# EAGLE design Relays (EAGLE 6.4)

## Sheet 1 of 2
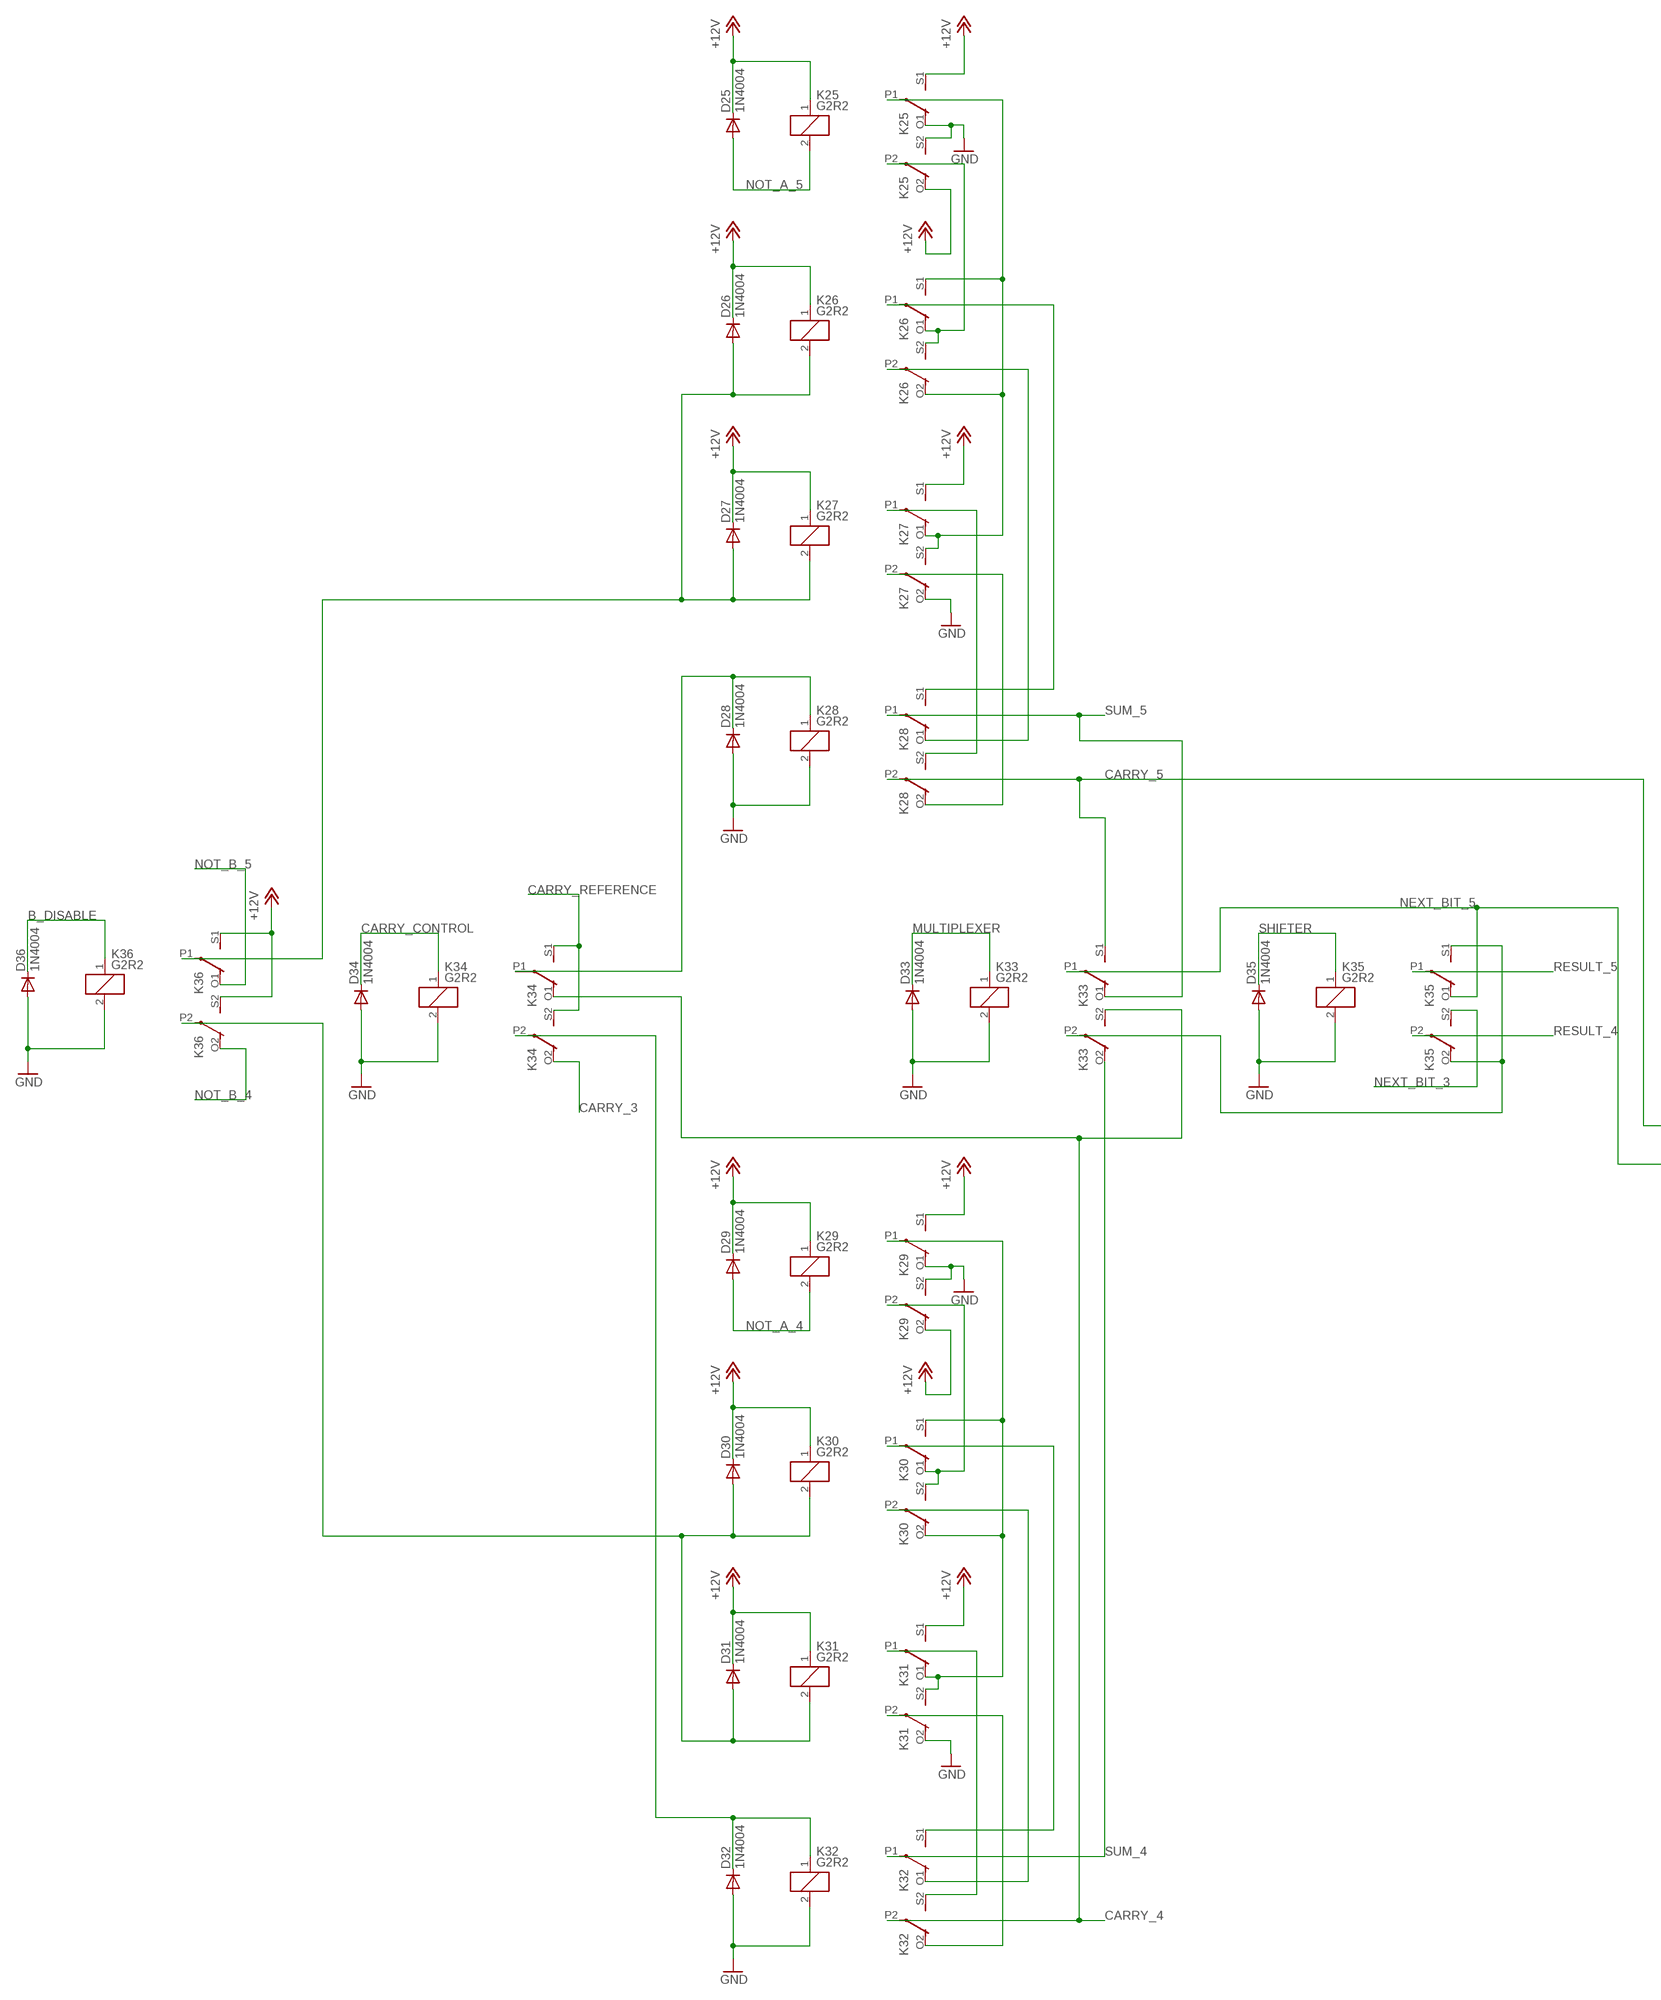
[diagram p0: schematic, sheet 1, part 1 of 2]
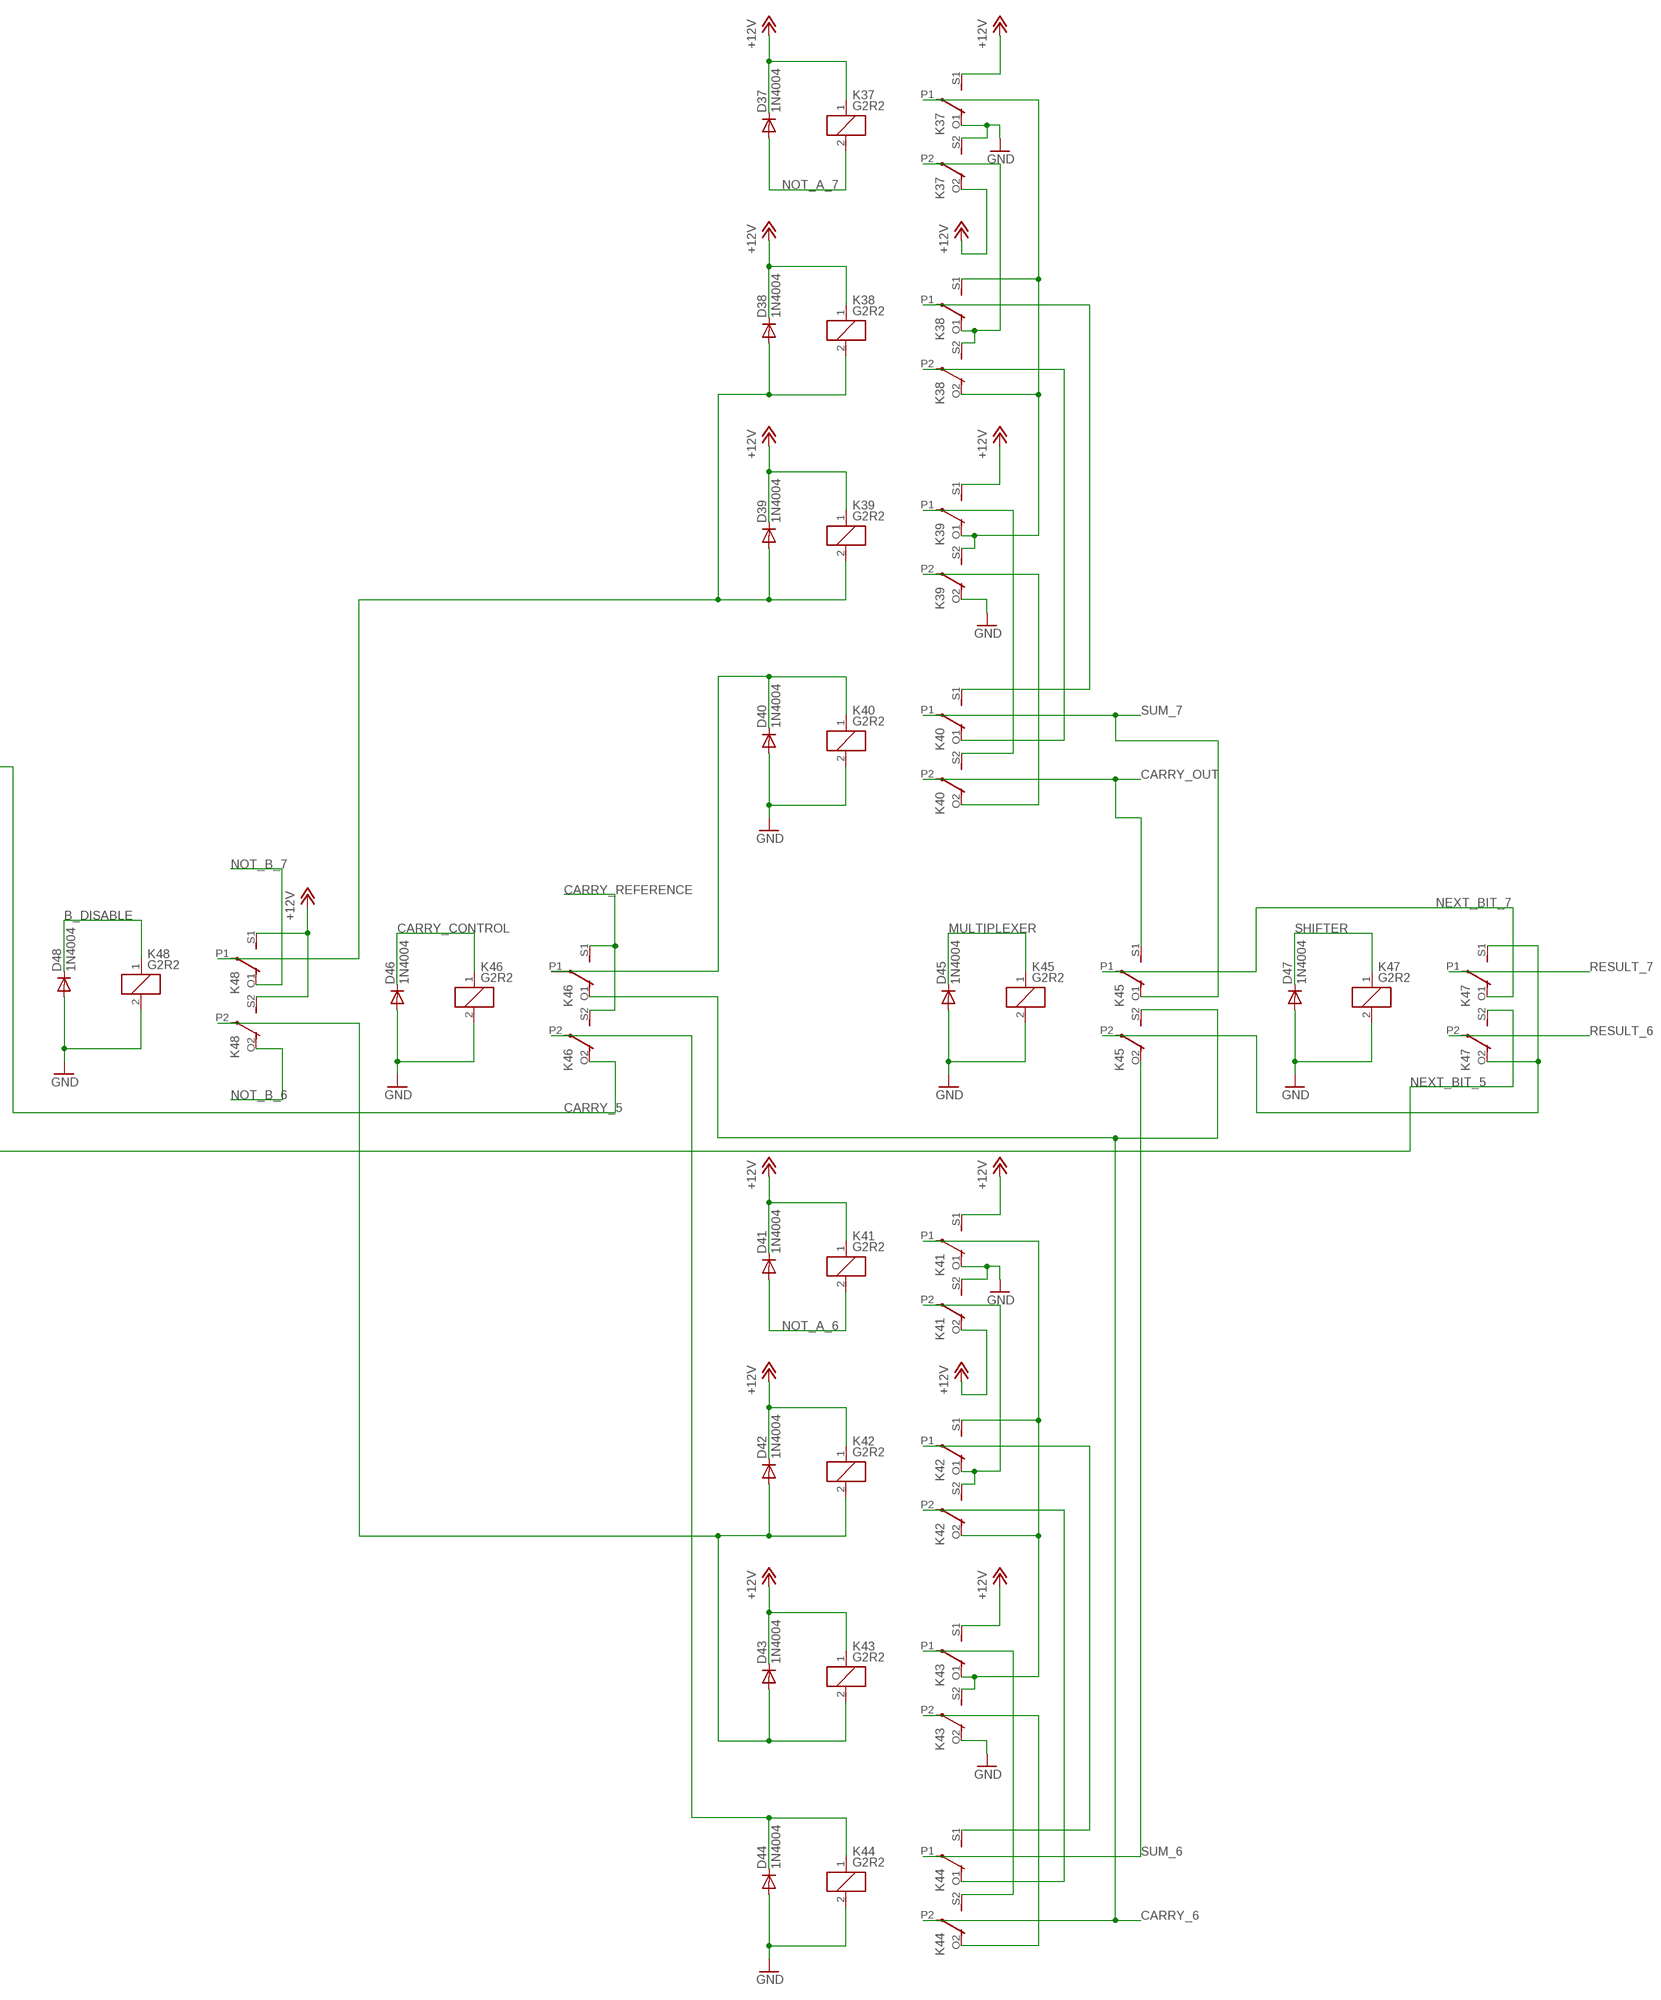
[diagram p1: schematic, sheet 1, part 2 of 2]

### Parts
D25  1N4004  [DO41-10]
D26  1N4004  [DO41-10]
D27  1N4004  [DO41-10]
D28  1N4004  [DO41-10]
D29  1N4004  [DO41-10]
D30  1N4004  [DO41-10]
D31  1N4004  [DO41-10]
D32  1N4004  [DO41-10]
D33  1N4004  [DO41-10]
D34  1N4004  [DO41-10]
D35  1N4004  [DO41-10]
D36  1N4004  [DO41-10]
D37  1N4004  [DO41-10]
D38  1N4004  [DO41-10]
D39  1N4004  [DO41-10]
D40  1N4004  [DO41-10]
D41  1N4004  [DO41-10]
D42  1N4004  [DO41-10]
D43  1N4004  [DO41-10]
D44  1N4004  [DO41-10]
D45  1N4004  [DO41-10]
D46  1N4004  [DO41-10]
D47  1N4004  [DO41-10]
D48  1N4004  [DO41-10]
K25  G2R2  [G2R2]
K26  G2R2  [G2R2]
K27  G2R2  [G2R2]
K28  G2R2  [G2R2]
K29  G2R2  [G2R2]
K30  G2R2  [G2R2]
K31  G2R2  [G2R2]
K32  G2R2  [G2R2]
K33  G2R2  [G2R2]
K34  G2R2  [G2R2]
K35  G2R2  [G2R2]
K36  G2R2  [G2R2]
K37  G2R2  [G2R2]
K38  G2R2  [G2R2]
K39  G2R2  [G2R2]
K40  G2R2  [G2R2]
K41  G2R2  [G2R2]
K42  G2R2  [G2R2]
K43  G2R2  [G2R2]
K44  G2R2  [G2R2]
K45  G2R2  [G2R2]
K46  G2R2  [G2R2]
K47  G2R2  [G2R2]
K48  G2R2  [G2R2]

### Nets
+12V [12V_Power]: D25.C D26.C D27.C D29.C D30.C D31.C D37.C D38.C D39.C D41.C D42.C D43.C K25.1 K25.O2(3:O) K25.S1(2:S) K26.1 K27.1 K27.S1(2:S) K29.1 K29.O2(3:O) K29.S1(2:S) K30.1 K31.1 K31.S1(2:S) K36.S1(2:S) K36.S2(3:S) K37.1 K37.O2(3:O) K37.S1(2:S) K38.1 K39.1 K39.S1(2:S) K41.1 K41.O2(3:O) K41.S1(2:S) K42.1 K43.1 K43.S1(2:S) K48.S1(2:S) K48.S2(3:S) ; also sheet 2
B_DISABLE [Relay_Interconnects]: D36.C D48.C K36.1 K48.1 ; also sheet 2
CARRY_3: K34.O2(3:O) ; also sheet 2
CARRY_4: K32.P2(3:P) K33.S2(3:S) K34.O1(2:O)
CARRY_5: K28.P2(3:P) K33.S1(2:S) K46.O2(3:O)
CARRY_6: K44.P2(3:P) K45.S2(3:S) K46.O1(2:O)
CARRY_CONTROL [Relay_Interconnects]: D34.C D46.C K34.1 K46.1 ; also sheet 2
CARRY_OUT [Relay_Interconnects]: K40.P2(3:P) K45.S1(2:S) ; also sheet 2
CARRY_REFERENCE [Relay_Interconnects]: K34.S1(2:S) K34.S2(3:S) K46.S1(2:S) K46.S2(3:S) ; also sheet 2
GND [Ground]: D28.A D32.A D33.A D34.A D35.A D36.A D40.A D44.A D45.A D46.A D47.A D48.A K25.O1(2:O) K25.S2(3:S) K27.O2(3:O) K28.2 K29.O1(2:O) K29.S2(3:S) K31.O2(3:O) K32.2 K33.2 K34.2 K35.2 K36.2 K37.O1(2:O) K37.S2(3:S) K39.O2(3:O) K40.2 K41.O1(2:O) K41.S2(3:S) K43.O2(3:O) K44.2 K45.2 K46.2 K47.2 K48.2 ; also sheet 2
MULTIPLEXER [Relay_Interconnects]: D33.C D45.C K33.1 K45.1 ; also sheet 2
N$37: D28.C K28.1 K34.P1(2:P)
N$38: K25.P2(3:P) K26.O1(2:O) K26.S2(3:S)
N$39: K25.P1(2:P) K26.O2(3:O) K26.S1(2:S) K27.O1(2:O) K27.S2(3:S)
N$40: K27.P2(3:P) K28.O2(3:O)
N$41: K27.P1(2:P) K28.S2(3:S)
N$42: K26.P2(3:P) K28.O1(2:O)
N$43: K26.P1(2:P) K28.S1(2:S)
N$44: D32.C K32.1 K34.P2(3:P)
N$45: K29.P2(3:P) K30.O1(2:O) K30.S2(3:S)
N$46: K29.P1(2:P) K30.O2(3:O) K30.S1(2:S) K31.O1(2:O) K31.S2(3:S)
N$47: K31.P2(3:P) K32.O2(3:O)
N$48: K31.P1(2:P) K32.S2(3:S)
N$49: K30.P2(3:P) K32.O1(2:O)
N$50: K30.P1(2:P) K32.S1(2:S)
N$51: D26.A D27.A K26.2 K27.2 K36.P1(2:P)
N$52: D30.A D31.A K30.2 K31.2 K36.P2(3:P)
N$53: K33.P2(3:P) K35.O2(3:O) K35.S1(2:S)
N$54: D40.C K40.1 K46.P1(2:P)
N$55: K37.P2(3:P) K38.O1(2:O) K38.S2(3:S)
N$56: K37.P1(2:P) K38.O2(3:O) K38.S1(2:S) K39.O1(2:O) K39.S2(3:S)
N$57: K39.P2(3:P) K40.O2(3:O)
N$58: K39.P1(2:P) K40.S2(3:S)
N$59: K38.P2(3:P) K40.O1(2:O)
N$60: K38.P1(2:P) K40.S1(2:S)
N$61: D44.C K44.1 K46.P2(3:P)
N$62: K41.P2(3:P) K42.O1(2:O) K42.S2(3:S)
N$63: K41.P1(2:P) K42.O2(3:O) K42.S1(2:S) K43.O1(2:O) K43.S2(3:S)
N$64: K43.P2(3:P) K44.O2(3:O)
N$65: K43.P1(2:P) K44.S2(3:S)
N$66: K42.P2(3:P) K44.O1(2:O)
N$67: K42.P1(2:P) K44.S1(2:S)
N$68: D38.A D39.A K38.2 K39.2 K48.P1(2:P)
N$69: D42.A D43.A K42.2 K43.2 K48.P2(3:P)
N$70: K45.P2(3:P) K47.O2(3:O) K47.S1(2:S)
NEXT_BIT_3 [Relay_Interconnects]: K35.S2(3:S) ; also sheet 2
NEXT_BIT_5: K33.P1(2:P) K35.O1(2:O) K47.S2(3:S)
NEXT_BIT_7 [Relay_Interconnects]: K45.P1(2:P) K47.O1(2:O) ; also sheet 2
NOT_A_4 [Relay_Interconnects]: D29.A K29.2 ; also sheet 2
NOT_A_5 [Relay_Interconnects]: D25.A K25.2 ; also sheet 2
NOT_A_6 [Relay_Interconnects]: D41.A K41.2 ; also sheet 2
NOT_A_7 [Relay_Interconnects]: D37.A K37.2 ; also sheet 2
NOT_B_4 [Relay_Interconnects]: K36.O2(3:O) ; also sheet 2
NOT_B_5 [Relay_Interconnects]: K36.O1(2:O) ; also sheet 2
NOT_B_6 [Relay_Interconnects]: K48.O2(3:O) ; also sheet 2
NOT_B_7 [Relay_Interconnects]: K48.O1(2:O) ; also sheet 2
RESULT_4 [Relay_Interconnects]: K35.P2(3:P) ; also sheet 2
RESULT_5 [Relay_Interconnects]: K35.P1(2:P) ; also sheet 2
RESULT_6 [Relay_Interconnects]: K47.P2(3:P) ; also sheet 2
RESULT_7 [Relay_Interconnects]: K47.P1(2:P) ; also sheet 2
SHIFTER [Relay_Interconnects]: D35.C D47.C K35.1 K47.1 ; also sheet 2
SUM_4: K32.P1(2:P) K33.O2(3:O)
SUM_5: K28.P1(2:P) K33.O1(2:O)
SUM_6: K44.P1(2:P) K45.O2(3:O)
SUM_7: K40.P1(2:P) K45.O1(2:O)

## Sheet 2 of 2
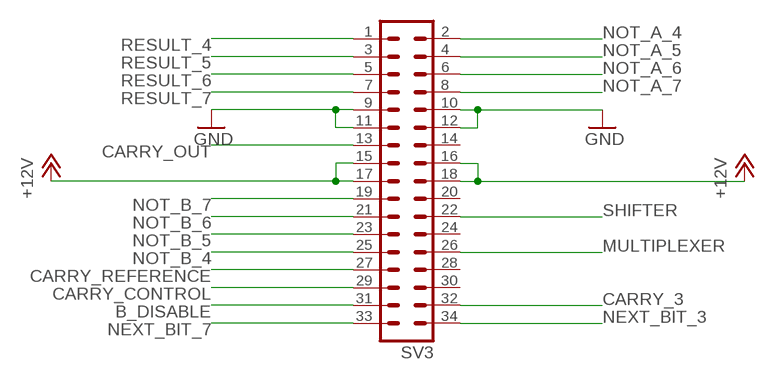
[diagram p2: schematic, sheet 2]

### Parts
SV3  ML34  [ML34]

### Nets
+12V [12V_Power]: SV3.15 SV3.16 SV3.17 SV3.18 ; also sheet 1
B_DISABLE [Relay_Interconnects]: SV3.31 ; also sheet 1
CARRY_3: SV3.32 ; also sheet 1
CARRY_CONTROL [Relay_Interconnects]: SV3.29 ; also sheet 1
CARRY_OUT [Relay_Interconnects]: SV3.13 ; also sheet 1
CARRY_REFERENCE [Relay_Interconnects]: SV3.27 ; also sheet 1
GND [Ground]: SV3.9 SV3.10 SV3.11 SV3.12 ; also sheet 1
MULTIPLEXER [Relay_Interconnects]: SV3.26 ; also sheet 1
NEXT_BIT_3 [Relay_Interconnects]: SV3.34 ; also sheet 1
NEXT_BIT_7 [Relay_Interconnects]: SV3.33 ; also sheet 1
NOT_A_4 [Relay_Interconnects]: SV3.2 ; also sheet 1
NOT_A_5 [Relay_Interconnects]: SV3.4 ; also sheet 1
NOT_A_6 [Relay_Interconnects]: SV3.6 ; also sheet 1
NOT_A_7 [Relay_Interconnects]: SV3.8 ; also sheet 1
NOT_B_4 [Relay_Interconnects]: SV3.25 ; also sheet 1
NOT_B_5 [Relay_Interconnects]: SV3.23 ; also sheet 1
NOT_B_6 [Relay_Interconnects]: SV3.21 ; also sheet 1
NOT_B_7 [Relay_Interconnects]: SV3.19 ; also sheet 1
RESULT_4 [Relay_Interconnects]: SV3.1 ; also sheet 1
RESULT_5 [Relay_Interconnects]: SV3.3 ; also sheet 1
RESULT_6 [Relay_Interconnects]: SV3.5 ; also sheet 1
RESULT_7 [Relay_Interconnects]: SV3.7 ; also sheet 1
SHIFTER [Relay_Interconnects]: SV3.22 ; also sheet 1
Unconnected: SV3.14 SV3.20 SV3.24 SV3.28 SV3.30

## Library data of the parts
D25-D48 = diode:1N4004: DIODE
K25-K48 = relay:G2R2: RELAY 2 x switch, Omron; MF: OMRON COMPONENTS USA; MPN: G2R-2-DC6; OC_FARNELL: unknown; OC_NEWARK: 89C5317
SV3 = con-harting-ml:ML34: HARTING; OC_FARNELL: unknown; OC_NEWARK: unknown

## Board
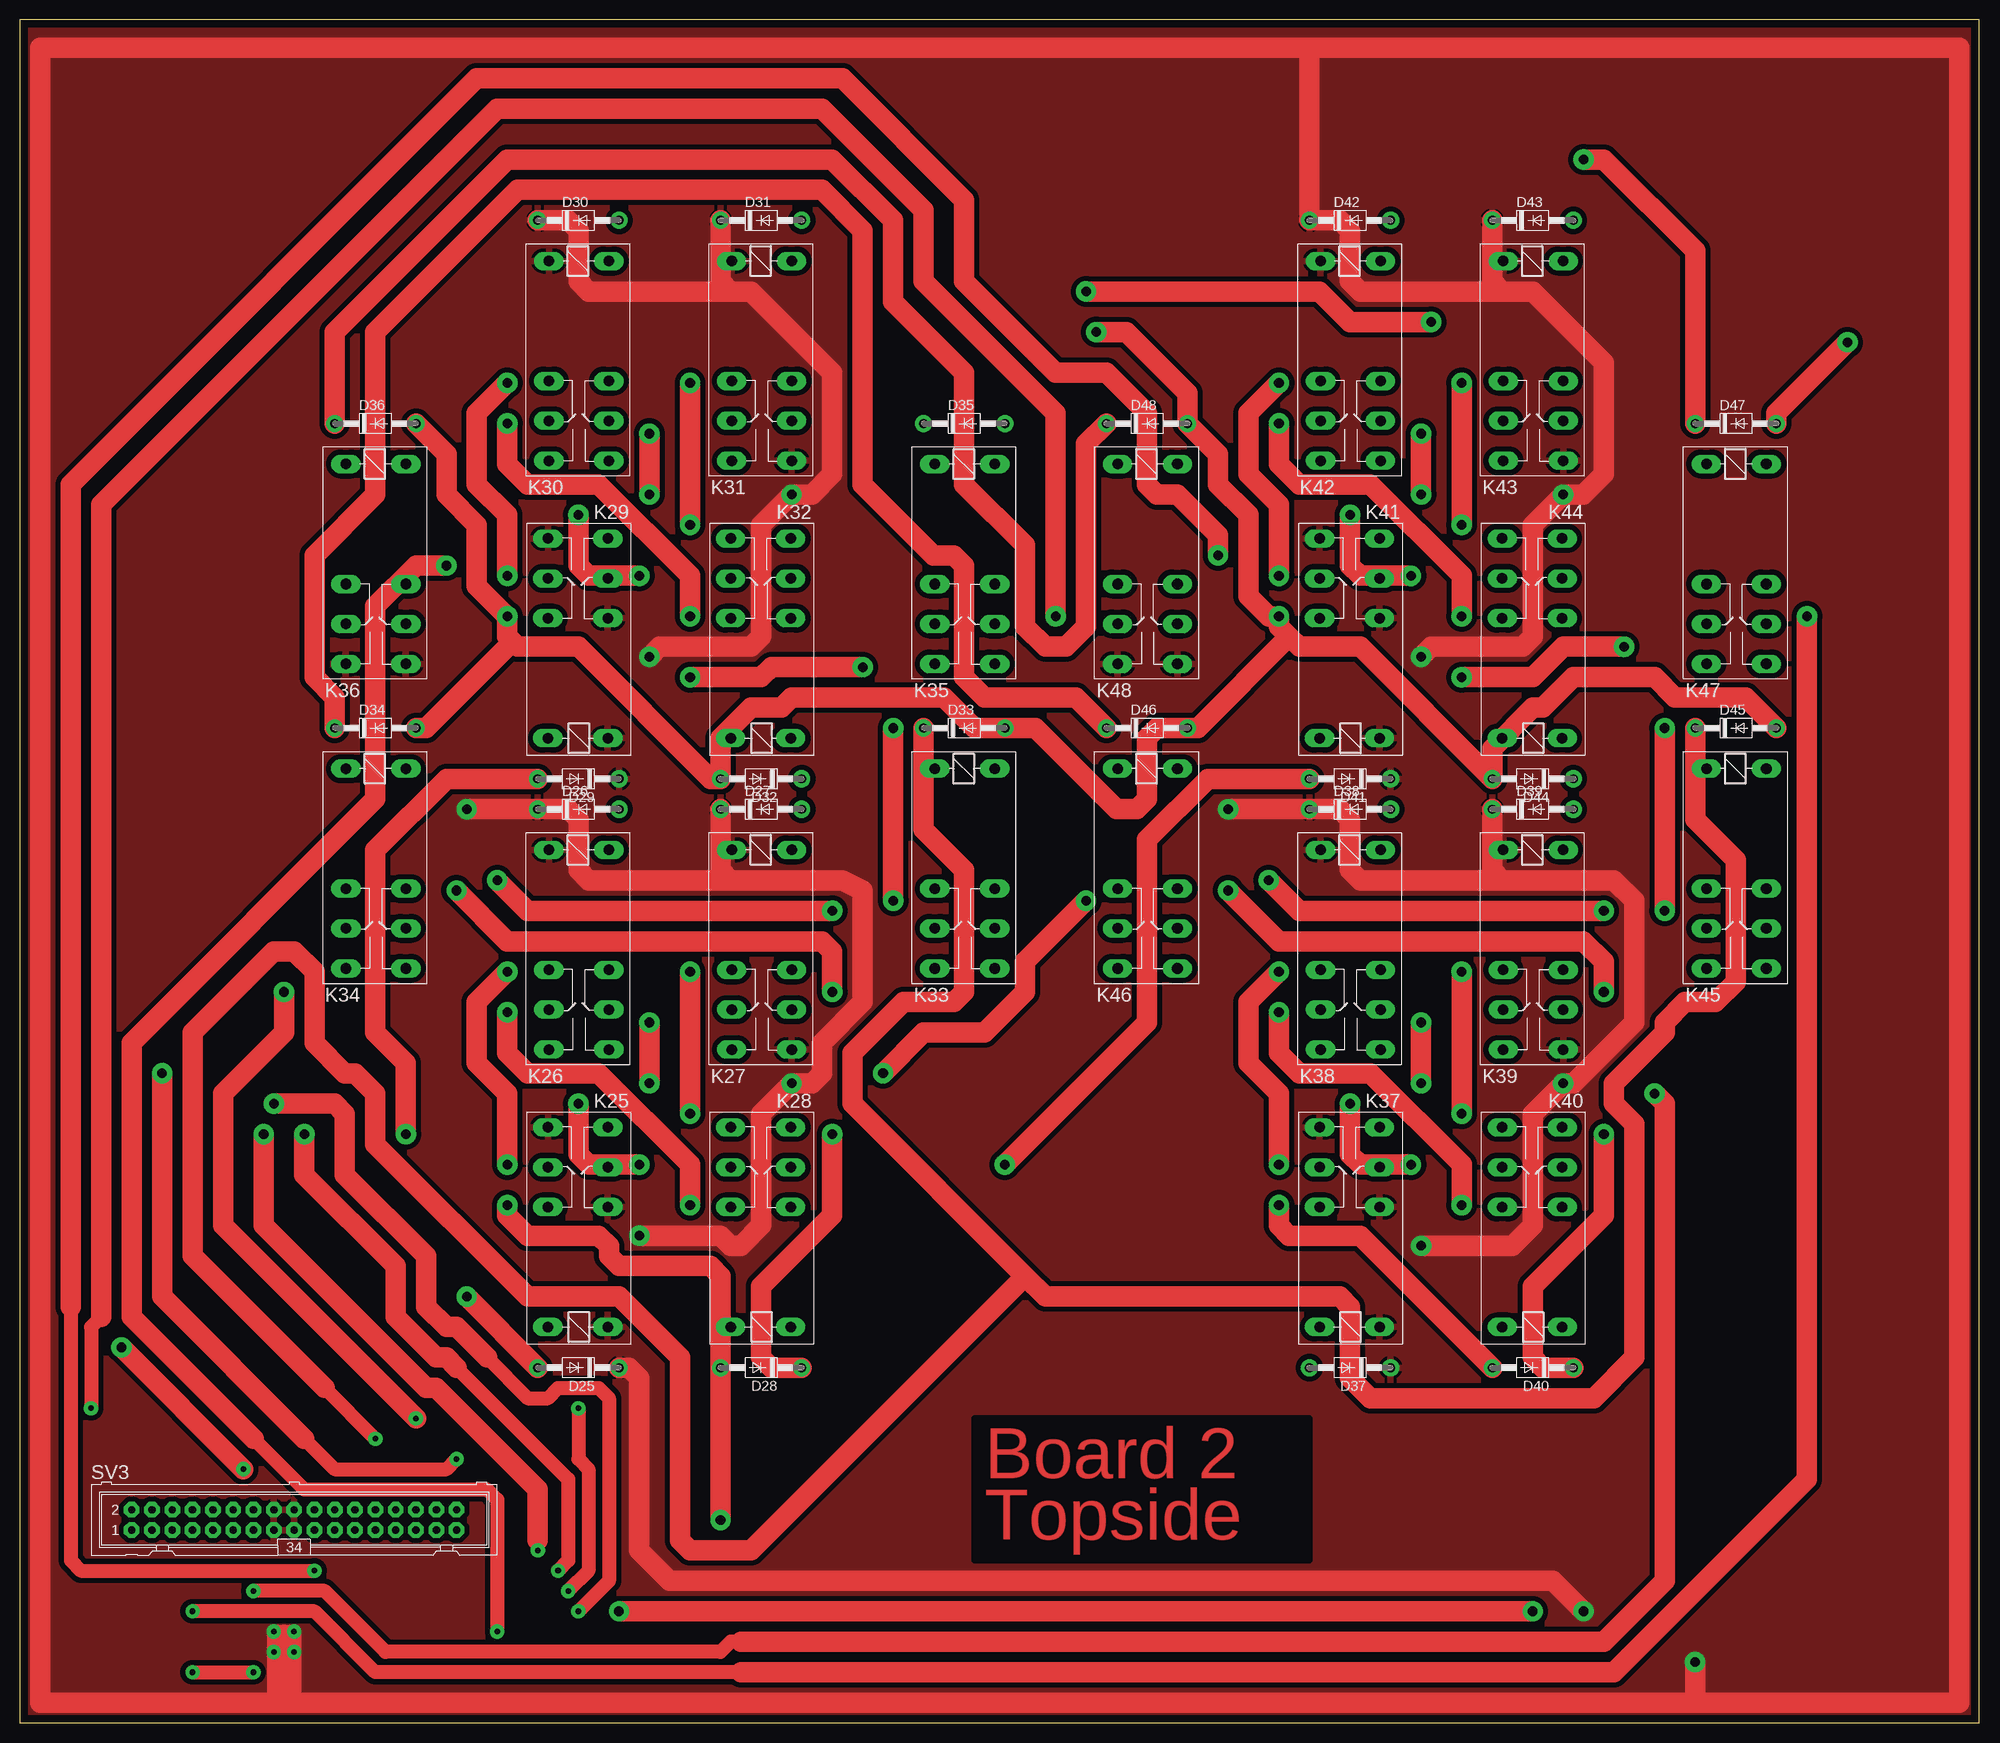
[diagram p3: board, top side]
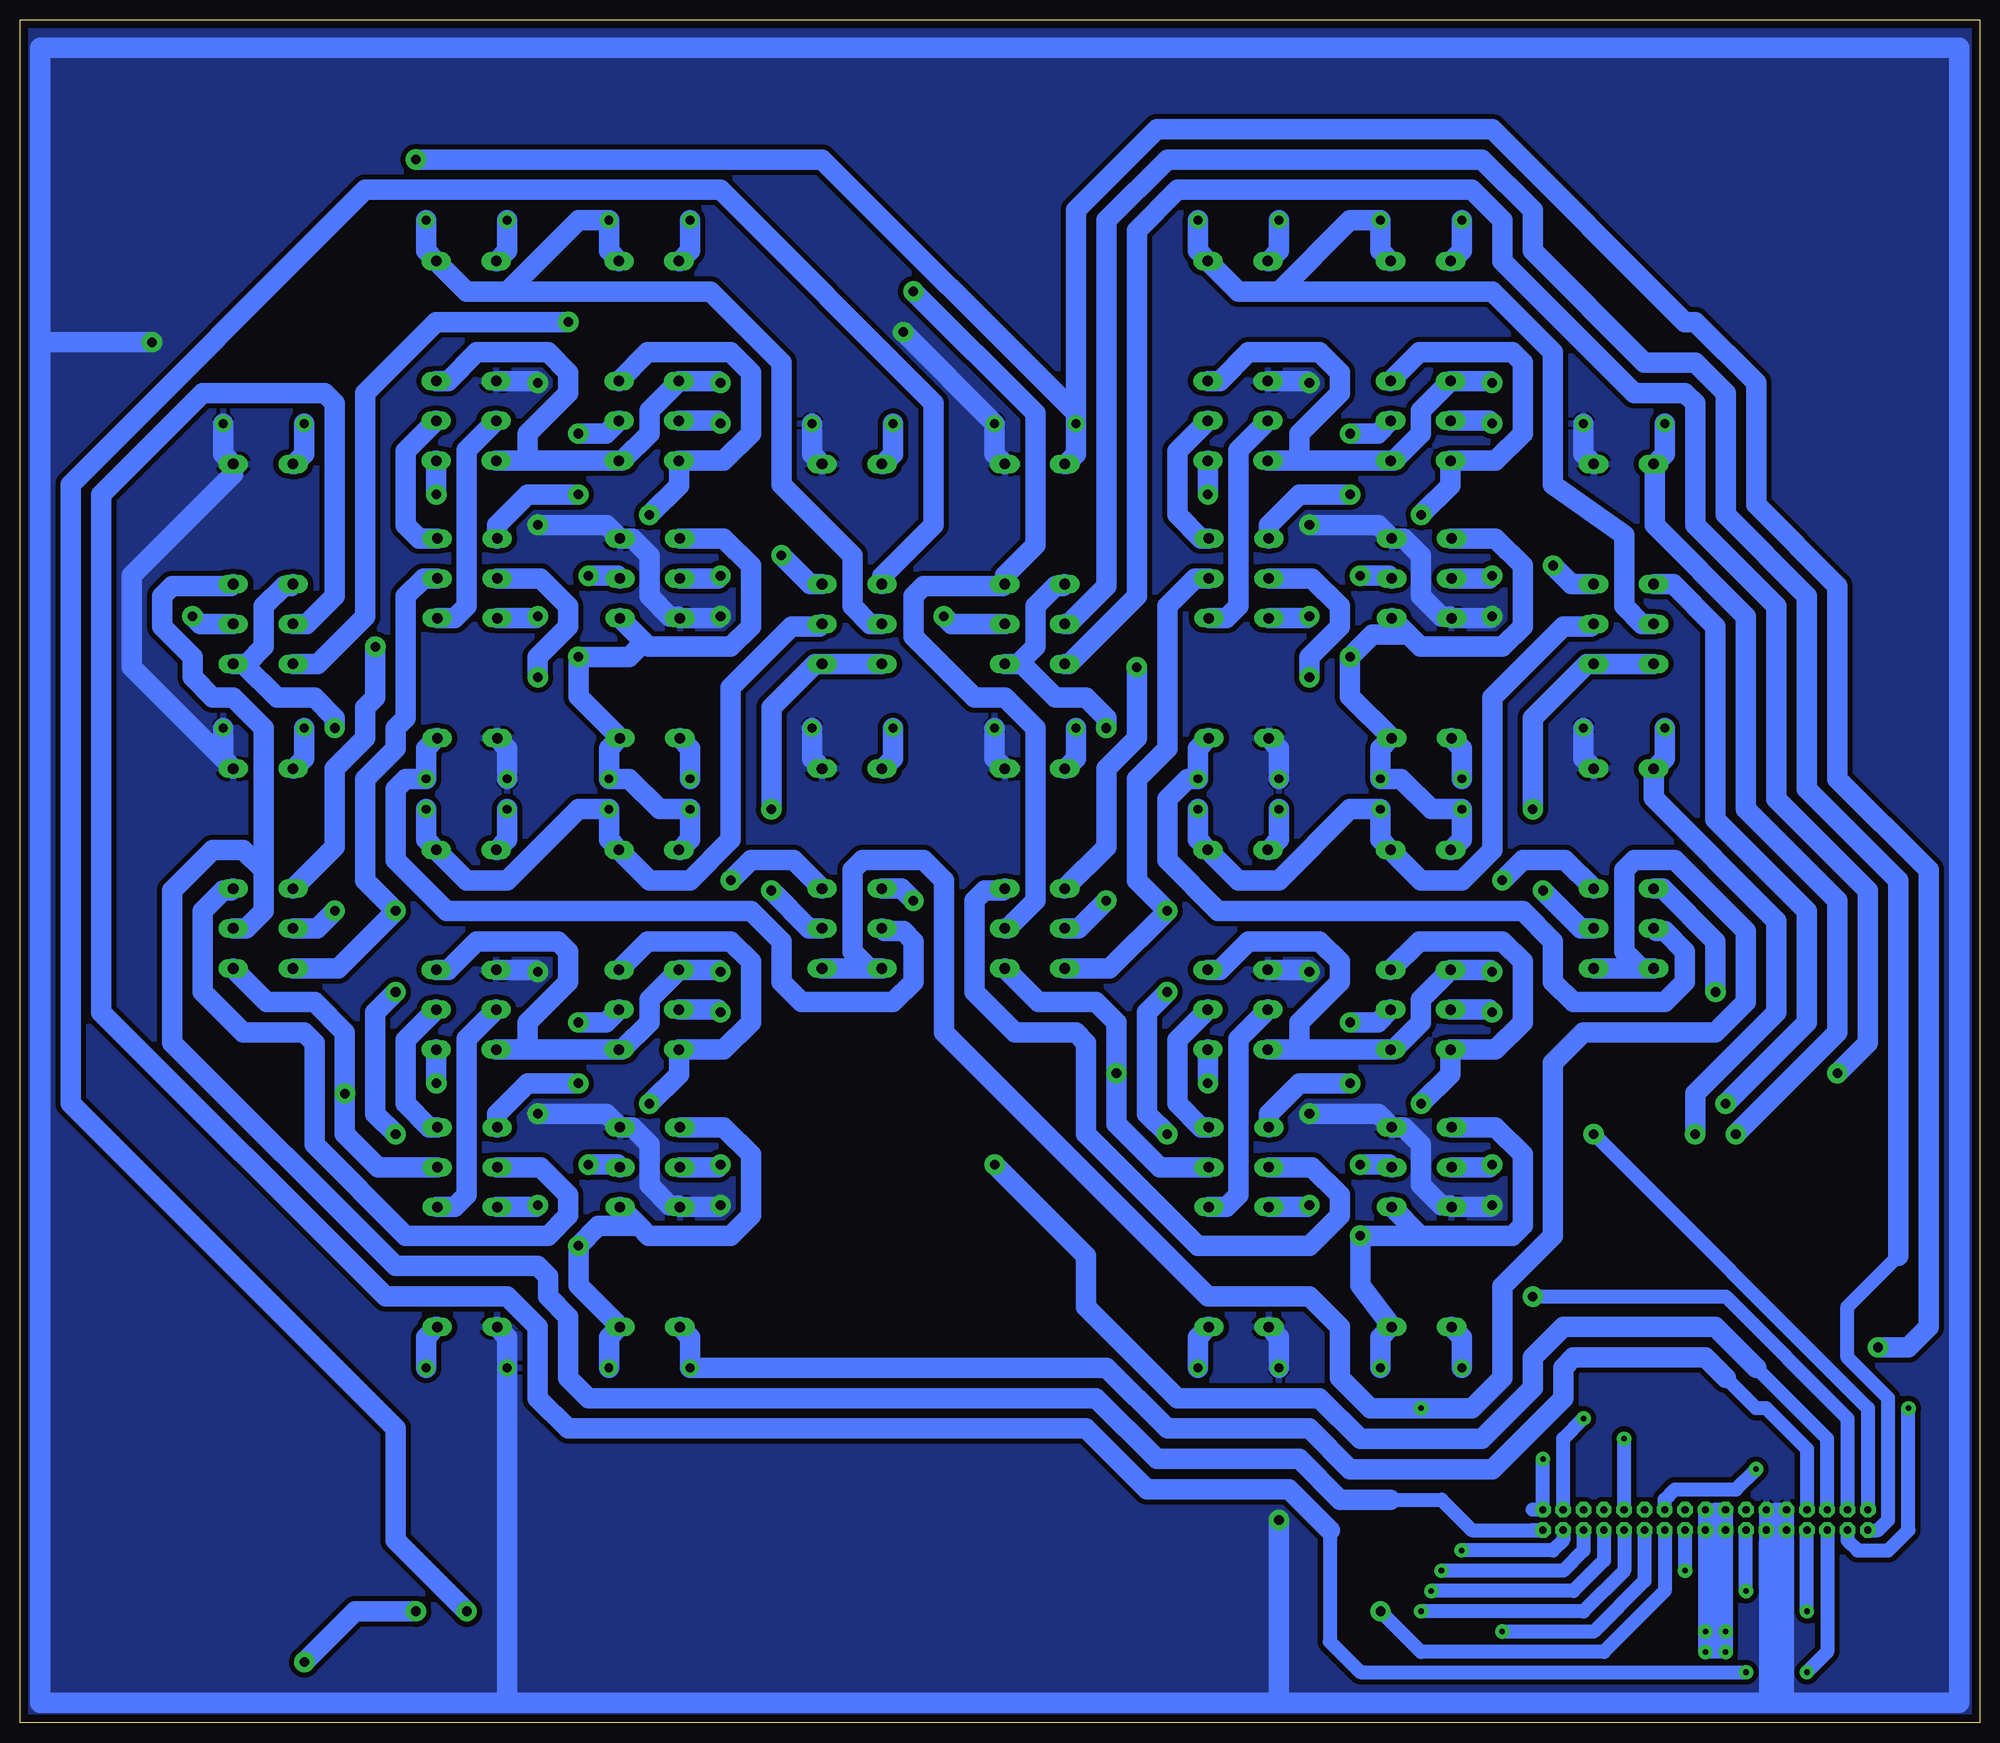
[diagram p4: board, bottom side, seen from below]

Size 245.09 x 213.03 mm. Coordinates in mm from the lower left corner, seen from the top.
Outline: 0,0 245.09,0 245.09,213.03 0,213.03 0,0
Copper layers (1*16): Top 0.035mm / dielectric 1.5mm / Bottom 0.035mm
Design rules "arm-rules-modified": minimum track width 20mil, minimum drill 24mil, track to track 25mil, track to pad 20mil, pad to pad 15mil, via to via 20mil, smd to smd 8mil, copper to edge 40mil, drill to drill 12mil, minimum pad ring 20mil, minimum via ring 20mil, stop-mask expansion 0mil, vias tented up to drill 0mil, thermal gap 15mil

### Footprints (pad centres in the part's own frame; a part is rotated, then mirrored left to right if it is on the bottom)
DO41-10 = drill 1.118: A 5.08,0; C -5.08,0
G2R2 = drill 1.321 long: 1 -2.54,-3.683; 2 -2.54,3.81; O1 12.471,3.81; O2 12.471,-3.683; P1 17.45,3.81; P2 17.45,-3.683; S1 22.454,3.81; S2 22.454,-3.683
ML34 = drill 0.914 octagon: 1 -20.32,-1.27; 2 -20.32,1.27; 3 -17.78,-1.27; 4 -17.78,1.27; 5 -15.24,-1.27; 6 -15.24,1.27; 7 -12.7,-1.27; 8 -12.7,1.27; 9 -10.16,-1.27; 10 -10.16,1.27; 11 -7.62,-1.27; 12 -7.62,1.27; 13 -5.08,-1.27; 14 -5.08,1.27; 15 -2.54,-1.27; 16 -2.54,1.27; 17 0,-1.27; 18 0,1.27; 19 2.54,-1.27; 20 2.54,1.27; 21 5.08,-1.27; 22 5.08,1.27; 23 7.62,-1.27; 24 7.62,1.27; 25 10.16,-1.27; 26 10.16,1.27; 27 12.7,-1.27; 28 12.7,1.27; 29 15.24,-1.27; 30 15.24,1.27; 31 17.78,-1.27; 32 17.78,1.27; 33 20.32,-1.27; 34 20.32,1.27

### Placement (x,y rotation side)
D25  69.85,44.45 180 top
D26  69.85,114.3 0 top
D27  92.71,114.3 0 top
D28  92.71,44.45 180 top
D29  69.85,118.11 180 top
D30  69.85,187.96 0 top
D31  92.71,187.96 0 top
D32  92.71,118.11 180 top
D33  118.11,124.46 0 top
D34  44.45,124.46 0 top
D35  118.11,162.56 0 top
D36  44.45,162.56 0 top
D37  166.37,44.45 180 top
D38  166.37,114.3 0 top
D39  189.23,114.3 0 top
D40  189.23,44.45 180 top
D41  166.37,118.11 180 top
D42  166.37,187.96 0 top
D43  189.23,187.96 0 top
D44  189.23,118.11 180 top
D45  214.63,124.46 0 top
D46  140.97,124.46 0 top
D47  214.63,162.56 0 top
D48  140.97,162.56 0 top
K25  69.85,52.07 90 top
K26  69.85,106.68 270 top
K27  92.71,106.68 270 top
K28  92.71,52.07 90 top
K29  69.85,125.73 90 top
K30  69.85,180.34 270 top
K31  92.71,180.34 270 top
K32  92.71,125.73 90 top
K33  118.11,116.84 270 top
K34  44.45,116.84 270 top
K35  118.11,154.94 270 top
K36  44.45,154.94 270 top
K37  166.37,52.07 90 top
K38  166.37,106.68 270 top
K39  189.23,106.68 270 top
K40  189.23,52.07 90 top
K41  166.37,125.73 90 top
K42  166.37,180.34 270 top
K43  189.23,180.34 270 top
K44  189.23,125.73 90 top
K45  214.63,116.84 270 top
K46  140.97,116.84 270 top
K47  214.63,154.94 270 top
K48  140.97,154.94 270 top
SV3  34.29,25.4 0 top

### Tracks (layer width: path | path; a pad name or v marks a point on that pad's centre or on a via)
+12V  (via drill 0.7 pad 1.78, 1.2 pad 2.54)
  Top 1.778: 31.75,2.54 v31.75,11.43 33.02,11.43 | 33.02,11.43 v34.29,11.43 v34.29,8.89 34.29,2.54 | 33.02,11.43 33.02,2.54
  Top 2.54: v175.26,59.69 186.69,59.69 189.23,62.23 189.23,76.2 v193.04,80.01 194.31,80.01 201.93,87.63 201.93,102.87 199.39,105.41 185.42,105.41 | 185.42,179.07 189.23,179.07 198.12,170.18 198.12,156.21 195.58,153.67 v193.04,153.67 189.23,149.86 189.23,135.89 187.96,134.62 176.53,134.62 v175.26,133.35 | 185.42,179.07 184.15,180.34 D43.C | 88.9,105.41 102.87,105.41 105.41,104.14 105.41,90.17 100.33,85.09 100.33,81.28 99.06,80.01 v96.52,80.01 92.71,76.2 92.71,62.23 90.17,59.69 88.9,59.69 87.63,60.96 v77.47,60.96 | 88.9,105.41 87.63,106.68 D27.C | 88.9,179.07 91.44,179.07 101.6,168.91 101.6,156.21 99.06,153.67 v96.52,153.67 92.71,149.86 92.71,135.89 91.44,134.62 80.01,134.62 v78.74,133.35 | 88.9,179.07 87.63,180.34 D31.C | 185.42,105.41 184.15,106.68 D39.C | 88.9,105.41 71.12,105.41 69.85,106.68 69.85,113.03 68.58,114.3 D26.C v55.88,114.3 | 88.9,179.07 71.12,179.07 69.85,180.34 69.85,186.69 68.58,187.96 D30.C | 185.42,105.41 167.64,105.41 166.37,106.68 166.37,113.03 165.1,114.3 D38.C v151.13,114.3 | 185.42,179.07 167.64,179.07 166.37,180.34 166.37,186.69 165.1,187.96 D42.C 161.29,209.55 | 209.55,2.54 242.57,2.54 242.57,209.55 161.29,209.55 | 209.55,2.54 34.29,2.54 33.02,2.54 31.75,2.54 2.54,2.54 2.54,209.55 161.29,209.55 | D25.C 76.2,44.45 77.47,43.18 77.47,21.59 81.28,17.78 191.77,17.78 v195.58,13.97 | v209.55,7.62 209.55,2.54
  Bottom 1.778: SV3.17 SV3.15 SV3.16 | SV3.16 33.02,26.67 | SV3.18 SV3.17 | SV3.17 SV3.16 | SV3.16 v31.75,11.43 | v31.75,11.43 v31.75,8.89 v34.29,8.89 | v34.29,8.89 v34.29,11.43 | v34.29,11.43 v31.75,11.43 | v31.75,11.43 33.02,10.16 | 33.02,10.16 v34.29,8.89 | v34.29,11.43 SV3.18 | SV3.18 33.02,26.67 | 33.02,26.67 33.02,10.16
  Bottom 2.54: D25.C 74.93,48.26 73.66,49.53 K25.1 77.47,54.74 v77.47,60.96 69.95,60.96 | D27.C 87.63,110.49 88.9,109.22 K27.1 | D30.C 64.77,184.15 66.04,182.88 K30.1 | D31.C 87.63,184.15 88.9,182.88 K31.1 | D37.C 171.45,48.26 170.18,49.53 K37.1 175.26,54.74 v175.26,59.69 172.78,62.17 167.68,62.17 | D39.C 184.15,110.49 185.42,109.22 K39.1 | D42.C 161.29,184.15 162.56,182.88 K42.1 | D43.C 184.15,184.15 185.42,182.88 K43.1 | K25.O2 69.95,60.96 | 69.95,60.96 58.42,60.96 57.15,62.23 57.15,71.12 60.55,74.52 K25.S1 | K41.O2 167.06,135.2 | 167.06,135.2 166.47,134.62 156.21,134.62 153.67,137.16 153.67,144.78 157.07,148.18 K41.S1 | K29.O2 71.46,136.13 | 71.46,136.13 69.95,134.62 59.69,134.62 57.15,137.16 57.15,144.78 60.55,148.18 K29.S1 | K37.O2 167.68,62.17 | 167.68,62.17 166.47,60.96 156.21,60.96 153.67,63.5 153.67,71.12 157.07,74.52 K37.S1 | K27.S1 v96.52,80.01 | K43.S1 v193.04,153.67 | K31.S1 v96.52,153.67 | K39.S1 v193.04,80.01 | 71.46,136.13 75.96,136.13 v78.74,133.35 78.74,128.4 K29.1 73.66,123.19 74.93,121.92 D29.C 72.39,118.11 68.58,114.3 D26.C 64.77,110.49 66.04,109.22 K26.1 | K36.S2 K36.S1 49.12,132.49 55.88,125.73 v55.88,114.3 | K48.S2 K48.S1 145.64,132.49 151.13,127 v151.13,114.3 | 167.06,135.2 168.91,133.35 v175.26,133.35 175.26,128.4 K41.1 170.18,123.19 171.45,121.92 D41.C 168.91,118.11 165.1,114.3 D38.C 161.29,110.49 162.56,109.22 K38.1 | v195.58,13.97 203.2,13.97 v209.55,7.62
  pour Top: 0,213.36 245.11,213.36 245.11,0 0,0
B_DISABLE  (via drill 0.7 pad 1.78, 1.2 pad 2.54)
  Top 1.778: 64.77,22.86 v64.77,21.59
  Top 2.54: D36.C 39.37,173.99 60.96,195.58 101.6,195.58 109.22,187.96 109.22,177.8 118.11,168.91 118.11,154.94 125.73,147.32 125.73,137.16 128.27,134.62 130.81,134.62 133.35,137.16 133.35,160.02 D48.C | v30.48,73.66 30.48,62.23 50.8,41.91 52.07,41.91 64.77,29.21 64.77,22.86
  Bottom 1.778: SV3.31 52.07,22.86 53.34,21.59 v64.77,21.59
  Bottom 2.54: D36.C 39.37,158.75 40.64,157.48 | D48.C 135.89,158.75 137.16,157.48 K48.1 | 40.64,157.48 40.64,149.86 29.21,138.43 29.21,114.3 17.78,102.87 17.78,86.36 v30.48,73.66 | 40.64,157.48 K36.1
CARRY_3  (via drill 0.7 pad 1.78, 1.2 pad 2.54)
  Top 2.54: v33.02,91.44 33.02,86.36 25.4,78.74 25.4,62.23 v49.53,38.1
  Bottom 1.778: SV3.32 52.07,35.56 v49.53,38.1
  Bottom 2.54: K34.O2 39.6,104.37 33.02,97.79 v33.02,91.44
CARRY_4  (via drill 1.2 pad 2.54)
  Top 2.54: v59.69,105.41 63.5,101.6 v101.6,101.6
  Bottom 2.54: K34.O1 51.84,107.95 57.15,107.95 v59.69,105.41 | K32.P2 98.12,143.18 101.6,139.7 101.6,121.92 105.41,118.11 105.41,105.41 v101.6,101.6 108.81,94.39 K33.S2
CARRY_5  (via drill 1.2 pad 2.54)
  Top 2.54: v107.95,81.28 113.03,86.36 120.65,86.36 125.73,91.44 125.73,95.25 v133.35,102.87
  Bottom 2.54: K28.P2 102.54,69.52 107.95,74.93 v107.95,81.28 107.95,87.63 110.49,90.17 117.7,90.17 K33.S1 | K46.O2 134.85,104.37 v133.35,102.87
CARRY_6  (via drill 1.2 pad 2.54)
  Top 2.54: v156.21,105.41 160.02,101.6 v198.12,101.6
  Bottom 2.54: K46.O1 148.36,107.95 153.67,107.95 v156.21,105.41 | K44.P2 194.64,143.18 196.85,140.97 196.85,125.73 198.12,124.46 198.12,121.92 201.93,118.11 201.93,105.41 v198.12,101.6 205.33,94.39 K45.S2
CARRY_CONTROL  (via drill 0.7 pad 1.78, 1.2 pad 2.54)
  Top 1.778: 54.61,44.45 68.58,30.48 68.58,20.32 v67.31,19.05
  Top 2.54: D34.C 39.37,128.27 36.83,130.81 36.83,146.05 44.45,153.67 44.45,173.99 62.23,191.77 100.33,191.77 105.41,186.69 105.41,154.94 114.3,146.05 116.84,146.05 118.11,144.78 118.11,130.81 120.65,128.27 132.08,128.27 D46.C | v35.56,73.66 35.56,68.58 46.99,57.15 46.99,50.8 52.07,45.72 53.34,45.72 54.61,44.45
  Bottom 1.778: SV3.29 49.53,21.59 52.07,19.05 v67.31,19.05
  Bottom 2.54: D34.C 39.37,120.65 40.64,119.38 K34.1 40.77,115.7 25.4,100.33 25.4,88.9 35.56,78.74 v35.56,73.66 | D46.C 135.89,120.65 137.16,119.38 K46.1
CARRY_OUT  (via drill 0.7 pad 1.78, 1.2 pad 2.54)
  Top 1.778: 90.17,10.16 88.9,10.16 87.63,8.89 45.72,8.89 38.1,16.51 v29.21,16.51
  Top 2.54: v204.47,78.74 205.74,77.47 205.74,17.78 198.12,10.16 132.08,10.16 129.54,10.16 90.17,10.16
  Bottom 1.778: v29.21,16.51 SV3.13
  Bottom 2.54: K40.P2 200.33,69.52 204.47,73.66 v204.47,78.74 204.47,86.36 208.28,90.17 214.22,90.17 K45.S1
CARRY_REFERENCE  (via drill 0.7 pad 1.78)
  Top 1.778: v69.85,39.37 69.85,33.02 71.12,31.75 71.12,19.05 v68.58,16.51
  Bottom 1.778: SV3.27 46.99,20.32 50.8,16.51 v68.58,16.51
  Bottom 2.54: K34.S1 K34.S2 42.32,94.39 44.45,96.52 44.45,106.68 43.18,107.95 38.1,107.95 29.21,99.06 29.21,90.17 33.02,86.36 49.53,86.36 53.34,82.55 53.34,60.96 59.69,54.61 59.69,43.18 63.5,39.37 v69.85,39.37 76.2,39.37 80.01,43.18 80.01,49.53 83.82,53.34 96.52,53.34 129.54,86.36 129.54,105.41 132.08,107.95 139.7,107.95 140.97,106.68 140.97,96.52 138.84,94.39 K46.S2 K46.S1
GND  (via drill 1.2 pad 2.54)
  Top 2.54: v83.82,76.2 v83.82,93.98 | v180.34,149.86 v180.34,167.64 | v83.82,149.86 v83.82,167.64 | v180.34,76.2 v180.34,93.98 | v60.96,64.77 60.96,63.5 63.5,60.96 72.39,60.96 73.66,59.69 73.66,58.42 74.93,57.15 86.36,57.15 87.63,55.88 D28.A v87.63,25.4 | 61.59,135.25 62.23,134.62 69.85,134.62 86.36,118.11 D32.A 87.63,123.19 91.44,127 95.25,127 96.52,128.27 115.57,128.27 119.38,124.46 D33.A 127,124.46 137.16,114.3 139.7,114.3 140.97,115.57 140.97,123.19 142.24,124.46 D46.A 147.32,124.46 158.75,135.89 | 61.59,135.25 60.96,135.89 v60.96,138.43 57.15,142.24 57.15,149.86 53.34,153.67 53.34,158.75 D36.A | 158.75,135.89 157.48,137.16 v157.48,138.43 156.21,138.43 153.67,140.97 153.67,151.13 149.86,154.94 149.86,158.75 D48.A 146.05,166.37 138.43,173.99 v134.62,173.99 | 158.75,135.89 160.02,134.62 167.64,134.62 D44.A 184.15,121.92 189.23,127 190.5,127 194.31,130.81 204.47,130.81 207.01,128.27 215.9,128.27 D45.A | D40.A 167.64,60.96 158.75,60.96 157.48,62.23 v157.48,64.77 | D34.A 50.8,124.46 61.59,135.25 | D47.A 219.71,163.83 v228.6,172.72
  Bottom 1.778: SV3.12 SV3.11 SV3.9 | SV3.9 SV3.10 | SV3.10 25.4,26.67 | 25.4,26.67 25.4,25.4 | 25.4,25.4 24.13,25.4 SV3.9 | SV3.10 24.13,2.54 | 26.67,2.54 SV3.12 | SV3.12 25.4,26.67 | 25.4,25.4 25.4,2.54
  Bottom 2.54: D36.A 49.53,158.75 K36.2 | D34.A 49.53,120.65 K34.2 | D33.A 123.19,120.65 K33.2 | K35.2 123.19,158.75 D35.A v134.62,173.99 | D48.A 146.05,158.75 K48.2 | D46.A 146.05,120.65 K46.2 | D45.A 219.71,120.65 K45.2 231.14,132.08 231.14,143.51 218.44,156.21 K47.2 219.71,158.75 D47.A | D28.A 87.63,48.26 K28.2 | D32.A 87.63,121.92 K32.2 | K40.2 184.15,48.26 D40.A 184.15,2.54 | D44.A 184.15,121.92 K44.2 | K27.O2 84.05,94.21 v83.82,93.98 | v60.96,64.77 61.19,64.54 K25.O1 66.27,64.77 67.31,64.77 69.85,67.31 69.85,72.39 71.98,74.52 K25.S2 75.21,76.2 v83.82,76.2 | K43.O2 180.57,167.87 v180.34,167.64 | v157.48,138.43 157.71,138.2 K41.O1 162.79,138.43 163.83,138.43 166.37,140.97 166.37,146.05 168.5,148.18 K41.S2 171.73,149.86 v180.34,149.86 | K31.O2 84.05,167.87 v83.82,167.64 | v60.96,138.43 61.19,138.2 K29.O1 66.27,138.43 67.31,138.43 69.85,140.97 69.85,146.05 71.98,148.18 K29.S2 75.21,149.86 v83.82,149.86 | K39.O2 180.57,94.21 v180.34,93.98 | v157.48,64.77 157.71,64.54 K37.O1 162.79,64.77 163.83,64.77 166.37,67.31 166.37,72.39 168.5,74.52 K37.S2 171.73,76.2 v180.34,76.2 | 184.15,2.54 242.57,2.54 242.57,172.72 | 184.15,2.54 87.63,2.54 | 87.63,2.54 26.67,2.54 25.4,2.54 24.13,2.54 2.54,2.54 2.54,209.55 242.57,209.55 242.57,172.72 | v228.6,172.72 242.57,172.72 | v87.63,25.4 87.63,2.54
  pour Bottom: 0,213.36 245.11,213.36 245.11,0 0,0
MULTIPLEXER  (via drill 0.7 pad 1.78)
  Top 1.778: v44.45,35.56 38.1,41.91
  Top 2.54: D33.C 113.03,111.76 118.11,106.68 118.11,91.44 116.84,90.17 110.49,90.17 104.14,83.82 104.14,77.47 125.73,55.88 | D45.C 209.55,113.03 214.63,107.95 214.63,92.71 212.09,90.17 208.28,90.17 205.74,87.63 205.74,86.36 199.39,80.01 199.39,77.47 201.93,74.93 201.93,45.72 196.85,40.64 168.91,40.64 166.37,43.18 166.37,52.07 165.1,53.34 128.27,53.34 125.73,55.88 | 38.1,41.91 21.59,58.42 21.59,86.36 31.75,96.52 34.29,96.52 36.83,93.98 36.83,85.09 40.64,81.28 41.91,81.28 44.45,78.74 44.45,72.39 63.5,53.34 74.93,53.34 82.55,45.72 82.55,22.86 83.82,21.59 91.44,21.59 125.73,55.88
  Bottom 1.778: SV3.26 v44.45,35.56
  Bottom 2.54: D33.C 113.03,120.65 114.3,119.38 K33.1 | D45.C 209.55,120.65 210.82,119.38 K45.1
N$3
  cutout Top (rank 2, no thermals): 119.38,38.1 161.29,38.1 161.29,20.32 119.38,20.32
N$37  (via drill 1.2 pad 2.54)
  Top 2.54: D28.C 93.98,44.45 92.71,45.72 92.71,54.61 101.6,63.5 v101.6,73.66 | v101.6,91.44 101.6,96.52 100.33,97.79 60.96,97.79 v54.61,104.14
  Bottom 2.54: D28.C 97.79,48.26 96.52,49.53 K28.1 | v101.6,73.66 104.14,76.2 104.14,88.9 v101.6,91.44 | K34.P1 49.86,99.39 v54.61,104.14
N$38  (via drill 1.2 pad 2.54)
  Top 2.54: v69.85,77.47 69.85,71.12 71.12,69.85 v77.47,69.85
  Bottom 2.54: K25.P2 73.86,69.85 v77.47,69.85 | v69.85,77.47 66.17,81.15 K26.S2 60.55,84.23 57.15,87.63 57.15,95.25 59.69,97.79 70.08,97.79 K26.O1
N$39  (via drill 1.2 pad 2.54)
  Top 2.54: v60.96,69.85 60.96,78.74 57.15,82.55 57.15,90.17 v60.96,93.98
  Bottom 2.54: K27.S2 85.09,84.23 | 85.09,84.23 K26.S1 73.25,84.23 69.85,87.63 69.85,90.53 K26.O2 61.19,94.21 v60.96,93.98 | K25.P1 61.29,69.52 v60.96,69.85 | K27.O1 95.02,94.21 91.44,97.79 82.55,97.79 80.01,95.25 80.01,92.71 85.09,87.63 85.09,84.23
N$40
  Bottom 2.54: K27.P2 92.71,85.55 92.71,66.04 94.21,64.54 K28.O2
N$41
  Bottom 2.54: K27.P1 100.33,85.42 100.33,77.47 97.38,74.52 K28.S2
N$42  (via drill 1.2 pad 2.54)
  Top 2.54: v83.82,64.77 83.82,69.85 72.39,81.28 63.5,81.28 60.96,83.82 v60.96,88.9
  Bottom 2.54: K28.O1 84.05,64.54 v83.82,64.77 | K26.P2 61.29,89.23 v60.96,88.9
N$43  (via drill 1.2 pad 2.54)
  Top 2.54: v78.74,80.01 v78.74,87.63
  Bottom 2.54: K26.P1 75.26,87.63 v78.74,87.63 | K28.S1 88.9,76.2 85.09,80.01 v78.74,80.01
N$44
  Bottom 2.54: K34.P2 40.44,99.06 39.37,99.06 36.83,96.52 36.83,92.71 39.37,90.17 50.8,90.17 53.34,92.71 53.34,97.79 57.15,101.6 95.25,101.6 101.6,107.95 101.6,115.57 99.06,118.11 D32.C 97.79,121.92 96.52,123.19 K32.1
N$45  (via drill 1.2 pad 2.54)
  Top 2.54: v69.85,151.13 69.85,144.78 71.12,143.51 v77.47,143.51
  Bottom 2.54: K29.P2 73.86,143.51 v77.47,143.51 | v69.85,151.13 66.17,154.81 K30.S2 60.55,157.89 57.15,161.29 57.15,170.18 58.42,171.45 70.08,171.45 K30.O1
N$46  (via drill 1.2 pad 2.54)
  Top 2.54: v60.96,143.51 60.96,151.13 57.15,154.94 57.15,163.83 v60.96,167.64
  Bottom 2.54: K31.S2 85.09,157.89 | 85.09,157.89 K30.S1 73.25,157.89 69.85,161.29 69.85,164.19 K30.O2 61.19,167.87 v60.96,167.64 | K29.P1 61.29,143.18 v60.96,143.51 | K31.O1 95.02,167.87 91.44,171.45 82.55,171.45 80.01,168.91 80.01,166.37 85.09,161.29 85.09,157.89
N$47
  Bottom 2.54: K31.P2 92.71,159.21 92.71,139.7 94.21,138.2 K32.O2
N$48
  Bottom 2.54: K31.P1 100.33,159.08 100.33,151.13 97.38,148.18 K32.S2
N$49  (via drill 1.2 pad 2.54)
  Top 2.54: v83.82,138.43 83.82,143.51 72.39,154.94 63.5,154.94 60.96,157.48 v60.96,162.56
  Bottom 2.54: K32.O1 84.05,138.2 v83.82,138.43 | K30.P2 61.29,162.89 v60.96,162.56
N$50  (via drill 1.2 pad 2.54)
  Top 2.54: v78.74,153.67 v78.74,161.29
  Bottom 2.54: K30.P1 75.26,161.29 v78.74,161.29 | K32.S1 88.9,149.86 85.09,153.67 v78.74,153.67
N$51
  Bottom 2.54: D27.A 97.79,110.49 K27.2 92.71,105.41 87.63,105.41 78.74,114.3 D26.A 74.93,110.49 K26.2 69.85,105.41 64.77,105.41 60.96,109.22 60.96,128.27 52.07,137.16 48.59,137.16 K36.P1
N$52
  Bottom 2.54: K30.2 74.93,184.15 D30.A 78.74,187.96 87.63,179.07 | D31.A 97.79,184.15 K31.2 92.71,179.07 87.63,179.07 | K36.P2 42.24,137.49 44.45,139.7 44.45,148.59 53.34,154.94 53.34,171.45 60.96,179.07 87.63,179.07
N$53  (via drill 1.2 pad 2.54)
  Top 2.54: v109.22,102.87 v109.22,124.46
  Bottom 2.54: K35.S1 120.24,132.49 | 120.24,132.49 118.11,134.62 118.11,139.7 115.57,142.24 114.66,142.24 K35.O2 | 120.24,132.49 119.79,132.49 115.57,128.27 111.76,128.27 109.22,125.73 v109.22,124.46 | K33.P2 112.7,99.39 v109.22,102.87
N$54  (via drill 1.2 pad 2.54)
  Top 2.54: D40.C 190.5,44.45 189.23,45.72 189.23,54.61 198.12,63.5 v198.12,73.66 | v198.12,91.44 198.12,95.25 195.58,97.79 157.48,97.79 v151.13,104.14
  Bottom 2.54: D40.C 194.31,48.26 193.04,49.53 K40.1 | v198.12,73.66 200.66,76.2 200.66,88.9 v198.12,91.44 | K46.P1 146.38,99.39 v151.13,104.14
N$55  (via drill 1.2 pad 2.54)
  Top 2.54: v166.37,77.47 166.37,71.12 167.64,69.85 v173.99,69.85
  Bottom 2.54: K37.P2 170.38,69.85 v173.99,69.85 | v166.37,77.47 162.69,81.15 K38.S2 157.07,84.23 153.67,87.63 153.67,95.25 156.21,97.79 166.6,97.79 K38.O1
N$56  (via drill 1.2 pad 2.54)
  Top 2.54: v157.48,69.85 157.48,78.74 153.67,82.55 153.67,90.17 v157.48,93.98
  Bottom 2.54: K37.P1 157.81,69.52 v157.48,69.85 | v157.48,93.98 157.71,94.21 K38.O2 166.37,90.53 166.37,87.63 169.77,84.23 K38.S1 K39.S2 182.47,84.23 181.61,85.09 181.61,87.63 176.53,92.71 176.53,96.52 177.8,97.79 187.96,97.79 191.54,94.21 K39.O1
N$57
  Bottom 2.54: K39.P2 189.23,85.55 189.23,66.04 190.73,64.54 K40.O2
N$58
  Bottom 2.54: K39.P1 196.85,85.42 196.85,77.47 193.9,74.52 K40.S2
N$59  (via drill 1.2 pad 2.54)
  Top 2.54: v180.34,64.77 180.34,69.85 168.91,81.28 160.02,81.28 157.48,83.82 v157.48,88.9
  Bottom 2.54: K40.O1 180.57,64.54 v180.34,64.77 | K38.P2 157.81,89.23 v157.48,88.9
N$60  (via drill 1.2 pad 2.54)
  Top 2.54: v175.26,80.01 v175.26,87.63
  Bottom 2.54: K38.P1 171.78,87.63 v175.26,87.63 | K40.S1 185.42,76.2 181.61,80.01 v175.26,80.01
N$61
  Bottom 2.54: K46.P2 136.96,99.06 134.62,99.06 133.35,97.79 133.35,92.71 135.89,90.17 147.32,90.17 149.86,92.71 149.86,97.79 153.67,101.6 191.77,101.6 198.12,107.95 198.12,116.84 196.85,118.11 D44.C 194.31,121.92 193.04,123.19 K44.1
N$62  (via drill 1.2 pad 2.54)
  Top 2.54: v166.37,151.13 166.37,144.78 167.64,143.51 v173.99,143.51
  Bottom 2.54: K41.P2 170.38,143.51 v173.99,143.51 | v166.37,151.13 162.69,154.81 K42.S2 157.07,157.89 153.67,161.29 153.67,168.91 156.21,171.45 166.6,171.45 K42.O1
N$63  (via drill 1.2 pad 2.54)
  Top 2.54: v157.48,143.51 157.48,152.4 153.67,156.21 153.67,163.83 v157.48,167.64
  Bottom 2.54: K43.S2 181.61,157.89 | 181.61,157.89 K42.S1 169.77,157.89 166.37,161.29 166.37,164.19 K42.O2 157.71,167.87 v157.48,167.64 | K41.P1 157.81,143.18 v157.48,143.51 | K43.O1 191.54,167.87 187.96,171.45 179.07,171.45 176.53,168.91 176.53,166.37 181.61,161.29 181.61,157.89
N$64
  Bottom 2.54: K43.P2 189.23,159.21 189.23,139.7 190.73,138.2 K44.O2
N$65
  Bottom 2.54: K43.P1 196.85,159.08 196.85,149.86 195.17,148.18 K44.S2
N$66  (via drill 1.2 pad 2.54)
  Top 2.54: v180.34,138.43 180.34,143.51 168.91,154.94 160.02,154.94 157.48,157.48 v157.48,162.56
  Bottom 2.54: K44.O1 180.57,138.2 v180.34,138.43 | K42.P2 157.81,162.89 v157.48,162.56
N$67  (via drill 1.2 pad 2.54)
  Top 2.54: v175.26,153.67 v175.26,161.29
  Bottom 2.54: K42.P1 171.78,161.29 v175.26,161.29 | K44.S1 185.42,149.86 181.61,153.67 v175.26,153.67
N$68
  Bottom 2.54: D39.A 194.31,110.49 K39.2 189.23,105.41 184.15,105.41 175.26,114.3 D38.A 171.45,110.49 K38.2 166.37,105.41 161.29,105.41 156.21,110.49 156.21,129.54 148.59,137.16 145.11,137.16 K48.P1
N$69
  Bottom 2.54: K42.2 171.45,184.15 D42.A 175.26,187.96 184.15,179.07 | D43.A 194.31,184.15 K43.2 189.23,179.07 184.15,179.07 | K48.P2 138.76,137.49 140.97,139.7 140.97,146.05 149.86,154.94 149.86,170.18 158.75,179.07 184.15,179.07
N$70  (via drill 1.2 pad 2.54)
  Top 2.54: v205.74,101.6 v205.74,124.46
  Bottom 2.54: K47.S1 217.17,132.49 | 217.17,132.49 216.76,132.49 214.63,134.62 214.63,139.7 212.09,142.24 211.18,142.24 K47.O2 | K45.P2 207.95,99.39 v205.74,101.6 | v205.74,124.46 205.74,125.73 208.28,128.27 212.95,128.27 217.17,132.49
NEXT_BIT_3  (via drill 0.7 pad 1.78, 1.2 pad 2.54)
  Top 1.778: 35.56,35.56 39.37,31.75 53.34,31.75 v54.61,33.02
  Top 2.54: v17.78,81.28 17.78,53.34 35.56,35.56
  Bottom 1.778: 55.88,26.67 SV3.34 v54.61,33.02
  Bottom 2.54: K35.S2 113.89,132.49 105.41,140.97 105.41,186.69 100.33,191.77 63.5,191.77 59.69,187.96 59.69,182.88 43.18,166.37 36.83,166.37 35.56,165.1 35.56,149.86 25.4,139.7 25.4,115.57 13.97,104.14 13.97,85.09 v17.78,81.28
NEXT_BIT_5  (via drill 1.2 pad 2.54)
  Top 2.54: v133.35,179.07 162.56,179.07 166.37,175.26 v176.53,175.26
  Bottom 2.54: K33.P1 121.59,99.39 118.11,102.87 118.11,124.46 121.92,128.27 125.73,128.27 133.35,135.89 133.35,140.97 132.08,142.24 122.15,142.24 K35.O1 121.92,143.51 118.11,147.32 118.11,163.83 v133.35,179.07 | K47.S2 207.87,132.49 201.93,138.43 201.93,166.37 193.04,175.26 v176.53,175.26
NEXT_BIT_7
  Bottom 1.778: 55.88,24.13 SV3.33 63.5,24.13 67.31,27.94 73.66,27.94
  Bottom 2.54: K45.P1 216.84,99.39 214.63,101.6 214.63,106.68 | 214.63,106.68 214.63,124.46 218.44,128.27 220.98,128.27 223.52,130.81 223.52,133.35 227.33,137.16 227.33,140.97 226.06,142.24 218.67,142.24 K47.O1 | 214.63,106.68 217.17,109.22 220.98,109.22 226.06,104.14 226.06,85.09 198.12,57.15 180.34,57.15 179.07,55.88 179.07,53.34 176.53,50.8 176.53,43.18 173.99,40.64 110.49,40.64 102.87,33.02 85.09,33.02 80.01,27.94 73.66,27.94
NOT_A_4  (via drill 1.2 pad 2.54)
  Top 2.54: D29.A 53.34,118.11 44.45,109.22 44.45,86.36 48.26,82.55 v48.26,73.66
  Bottom 1.778: v48.26,73.66 13.97,39.37 SV3.2
  Bottom 2.54: D29.A 64.77,121.92 K29.2
NOT_A_5  (via drill 1.2 pad 2.54)
  Top 2.54: D25.A v55.88,53.34
  Bottom 1.778: v55.88,53.34 31.75,53.34 16.51,38.1 SV3.4
  Bottom 2.54: D25.A 64.77,48.26 K25.2
NOT_A_6  (via drill 1.2 pad 2.54)
  Top 2.54: D41.A 148.59,118.11 140.97,110.49 140.97,87.63 v123.19,69.85
  Bottom 1.778: SV3.6 19.05,35.56 27.94,44.45
  Bottom 2.54: D41.A 161.29,121.92 K41.2 | v123.19,69.85 111.76,58.42 111.76,52.07 100.33,40.64 82.55,40.64 77.47,35.56 62.23,35.56 55.88,41.91 55.88,45.72 52.07,49.53 33.02,49.53 27.94,44.45
NOT_A_7
  Bottom 1.778: SV3.8 21.59,34.29 26.67,39.37 27.94,39.37 31.75,43.18
  Bottom 2.54: K37.2 161.29,48.26 D37.A 109.22,44.45 101.6,36.83 83.82,36.83 78.74,31.75 60.96,31.75 52.07,40.64 52.07,44.45 50.8,45.72 34.29,45.72 31.75,43.18
NOT_B_4  (via drill 0.7 pad 1.78, 1.2 pad 2.54)
  Top 1.778: 58.42,45.72 63.5,40.64 66.04,40.64 67.31,41.91 72.39,41.91 73.66,40.64 73.66,17.78 v69.85,13.97
  Top 2.54: v31.75,77.47 39.37,77.47 40.64,76.2 40.64,68.58 50.8,58.42 50.8,52.07 53.34,49.53 54.61,49.53 58.42,45.72
  Bottom 1.778: SV3.25 44.45,19.05 49.53,13.97 v69.85,13.97
  Bottom 2.54: K36.O2 38.33,142.47 33.02,137.16 33.02,113.03 21.59,101.6 21.59,87.63 v31.75,77.47
NOT_B_5  (via drill 0.7 pad 1.78, 1.2 pad 2.54)
  Top 1.778: v59.69,11.43 59.69,27.94 58.42,29.21 35.56,29.21 29.21,35.56
  Top 2.54: v53.34,144.78 49.53,144.78 44.45,139.7 44.45,115.57 13.97,85.09 13.97,50.8 29.21,35.56
  Bottom 1.778: SV3.23 41.91,17.78 48.26,11.43 v59.69,11.43
  Bottom 2.54: K36.O1 51.03,142.47 v53.34,144.78
NOT_B_6  (via drill 1.2 pad 2.54)
  Top 2.54: v189.23,13.97 v74.93,13.97
  Bottom 1.778: SV3.21 39.37,16.51 46.99,8.89 69.85,8.89 v74.93,13.97
  Bottom 2.54: K48.O2 137.29,143.38 130.81,149.86 130.81,165.1 157.48,191.77 201.93,191.77 238.76,154.94 238.76,77.47 198.12,36.83 198.12,22.86 v189.23,13.97
NOT_B_7  (via drill 0.7 pad 1.78, 1.2 pad 2.54)
  Top 1.778: 6.35,52.07 6.35,20.32 7.62,19.05 v36.83,19.05
  Top 2.54: v149.86,146.05 149.86,148.59 144.78,153.67 142.24,153.67 140.97,154.94 140.97,163.83 135.89,168.91 129.54,168.91 118.11,180.34 118.11,190.5 102.87,205.74 57.15,205.74 6.35,154.94 6.35,52.07
  Bottom 1.778: SV3.19 v36.83,19.05
  Bottom 2.54: K48.O1 146.28,142.47 v149.86,146.05
RESULT_4
  Bottom 1.778: SV3.1 12.7,24.13 11.43,25.4 11.43,40.64 16.51,45.72 16.51,52.07 10.16,58.42
  Bottom 2.54: K35.P2 113.97,137.49 109.22,142.24 109.22,187.96 101.6,195.58 62.23,195.58 55.88,189.23 55.88,184.15 41.91,170.18 35.56,170.18 31.75,166.37 31.75,151.13 21.59,140.97 21.59,116.84 10.16,105.41 10.16,58.42
RESULT_5  (via drill 0.7 pad 1.78, 1.2 pad 2.54)
  Top 1.778: 10.16,50.8 8.89,49.53 v8.89,39.37
  Top 2.54: v129.54,138.43 129.54,163.83 113.03,180.34 113.03,189.23 100.33,201.93 59.69,201.93 10.16,152.4 10.16,50.8
  Bottom 1.778: SV3.3 16.51,22.86 15.24,21.59 11.43,21.59 8.89,24.13 v8.89,39.37
  Bottom 2.54: K35.P1 128.6,137.49 v129.54,138.43
RESULT_6  (via drill 0.7 pad 1.78)
  Top 1.778: v21.59,6.35 v29.21,6.35
  Bottom 1.778: 81.28,24.13 81.28,10.16 77.47,6.35 v29.21,6.35 | SV3.5 19.05,8.89 v21.59,6.35
  Bottom 2.54: K47.P2 209.22,137.49 205.74,140.97 205.74,165.1 207.01,166.37 222.25,166.37 234.95,153.67 234.95,88.9 199.39,53.34 184.15,53.34 180.34,49.53 180.34,40.64 176.53,36.83 111.76,36.83 104.14,29.21 86.36,29.21 81.28,24.13
RESULT_7  (via drill 0.7 pad 1.78, 1.2 pad 2.54)
  Top 1.778: 90.17,6.35 44.45,6.35 36.83,13.97 v21.59,13.97
  Top 2.54: v223.52,138.43 223.52,30.48 199.39,6.35 134.62,6.35 132.08,6.35 90.17,6.35
  Bottom 1.778: v21.59,13.97 SV3.7
  Bottom 2.54: K47.P1 222.58,137.49 v223.52,138.43
SHIFTER  (via drill 0.7 pad 1.78, 1.2 pad 2.54)
  Top 2.54: v195.58,195.58 198.12,195.58 209.55,184.15 D47.C | v12.7,46.99 v27.94,31.75
  Bottom 1.778: SV3.22 39.37,27.94 38.1,29.21 30.48,29.21 v27.94,31.75
  Bottom 2.54: D35.C 113.03,158.75 114.3,157.48 K35.1 | D47.C 209.55,158.75 210.82,157.48 K47.1 | D35.C 113.03,189.23 102.87,199.39 60.96,199.39 36.83,175.26 35.56,175.26 27.94,167.64 27.94,152.4 17.78,142.24 17.78,118.11 6.35,106.68 6.35,49.53 8.89,46.99 v12.7,46.99 | D35.C 113.03,163.83 144.78,195.58 v195.58,195.58
SUM_4  (via drill 1.2 pad 2.54)
  Top 2.54: v83.82,130.81 92.71,130.81 93.98,132.08 v105.41,132.08
  Bottom 2.54: K32.P1 83.49,143.18 80.01,139.7 80.01,137.16 83.82,133.35 v83.82,130.81 | K33.O2 109.22,109.58 109.22,119.38 105.41,123.19 v105.41,132.08
SUM_5
  Bottom 2.54: K28.P1 83.49,69.52 80.01,66.04 80.01,63.5 83.82,59.69 97.79,59.69 111.76,73.66 111.76,85.09 113.03,86.36 120.65,86.36 125.73,91.44 125.73,102.87 124.46,104.14 122.15,104.14 K33.O1
SUM_6  (via drill 1.2 pad 2.54)
  Top 2.54: v180.34,130.81 189.23,130.81 193.04,134.62 v200.66,134.62
  Bottom 2.54: K44.P1 180.01,143.18 176.53,139.7 176.53,137.16 180.34,133.35 v180.34,130.81 | K45.O2 205.74,109.58 205.74,119.38 201.93,123.19 201.93,127 200.66,128.27 v200.66,134.62
SUM_7
  Bottom 2.54: K40.P1 180.01,69.52 176.53,66.04 176.53,63.5 179.07,60.96 196.85,60.96 208.28,72.39 208.28,85.09 209.55,86.36 217.17,86.36 222.25,91.44 222.25,101.6 219.71,104.14 218.67,104.14 K45.O1

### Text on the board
Top: Board 2 / Topside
